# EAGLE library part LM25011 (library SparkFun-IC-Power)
The LM25011 constant on-time step-down switching regulator features all the functions needed to implement a low-cost, efficient, buck bias regulator capable of supplying up to 2 A of load current. This high-voltage regulator contains an N-Channel Buck switch, a startup regulator, current limit detection, and internal ripple control.
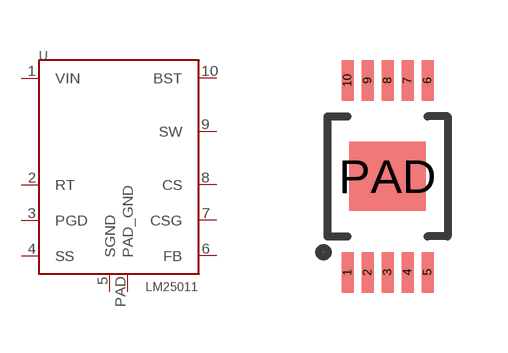
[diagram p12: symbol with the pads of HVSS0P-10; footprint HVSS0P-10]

Designator prefix U

## LM25011 (PROD_ID: IC-12528)  [HVSS0P-10]
1  VIN
2  RT
3  PGD
4  SS
5  SGND
6  FB
7  CSG
8  CS
9  SW
10  BST
PAD  PAD_GND

## Footprint HVSS0P-10 (pad centres in mm)
smd 0.3 x 1.02: 1 -1,-2.4; 2 -0.5,-2.4; 3 0,-2.4; 4 0.5,-2.4; 5 1,-2.4; 6 1,2.4; 7 0.5,2.4; 8 0,2.4; 9 -0.5,2.4; 10 -1,2.4
smd 1.905 x 1.727: PAD 0,0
